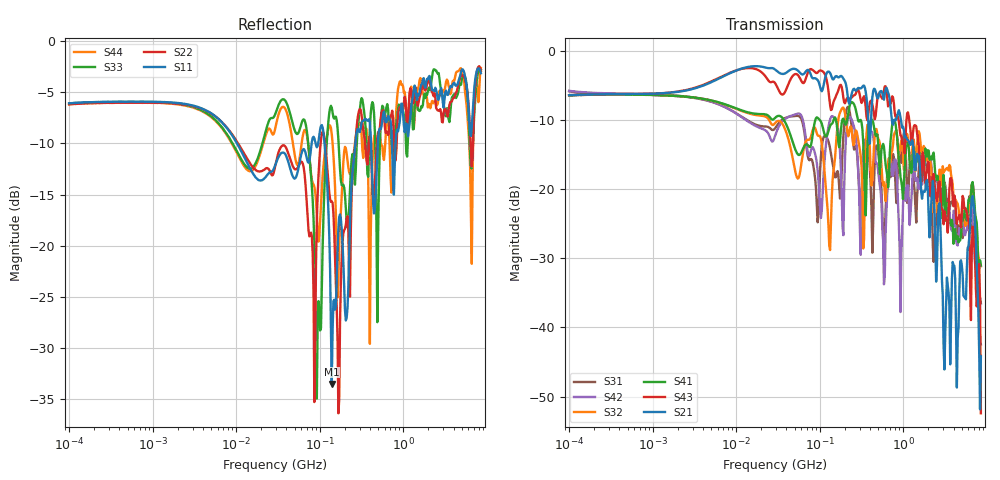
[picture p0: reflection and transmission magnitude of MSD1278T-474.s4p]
# MHz S MA R 50
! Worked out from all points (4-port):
!   498 points, 100 kHz to 8.5 GHz, reference 50 ohm
!   strongest paths, dB at 100 kHz, 1.698 MHz, 29.49 MHz, 500.7 MHz, 8.5 GHz:
!     S21: -6.3, -6.0, -2.7, -6.8, -44.2
!     S43: -6.3, -5.9, -4.7, -6.2, -52.4
!     S41: -6.4, -6.4, -9.6, -13.2, -31.0
!     S32: -6.4, -6.4, -10.3, -12.6, -31.1
!     S42: -5.7, -6.4, -12.1, -17.4, -42.4
!     S31: -5.8, -6.4, -11.1, -14.3, -36.5
!   lowest |S11| = -33.5 dB at 139.4 MHz (marker M1), VSWR 1.04, Z = 49.2 - j1.95 ohm
!   |S11| at or under -10 dB: 10.23 MHz to 80.11 MHz (69.88 MHz wide, 155 % of centre); 114.2 MHz to 267.3 MHz (153.1 MHz wide, 80.3 % of centre); 411.1 MHz to 496.6 MHz (85.5 MHz wide, 18.8 % of centre)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
0.1  0.4965 9.5  0.4816 10.7  0.5139 -10.4  0.4796 -170.7
     0.4816 10.7  0.491 9.5  0.4794 -170.6  0.5185 -10.4
     0.5139 -10.4  0.4794 -170.6  0.4954 9.6  0.4817 10.6
     0.4796 -170.7  0.5185 -10.4  0.4817 10.6  0.4895 9.7
37.91146  0.2831 -18.0  0.6897 -8.1  0.328 143.2  0.3131 -14.9
          0.6897 -8.1  0.3081 -21.9  0.2793 -13.7  0.3218 140.6
          0.328 143.2  0.2793 -13.7  0.516 -21.2  0.5011 -2.1
          0.3131 -14.9  0.3218 140.6  0.5011 -2.1  0.4724 -22.7
94.51579  0.307 -42.1  0.6194 -27.6  0.05783 27.1  0.3304 61.7
          0.6194 -27.6  0.1778 51.5  0.2463 17.5  0.1368 -51.7
          0.05783 27.1  0.2463 17.5  0.04302 2.5  0.7036 -23.4
          0.3304 61.7  0.1368 -51.7  0.7036 -23.4  0.1177 -47.5
139.353  0.02113 -110.7  0.6498 -33.4  0.1669 -10.5  0.2983 27.8
         0.6498 -33.4  0.1651 -55.2  0.0868 77.1  0.3393 27.6
         0.1669 -10.5  0.0868 77.1  0.4728 -13.7  0.3785 -34.4
         0.2983 27.8  0.3393 27.6  0.3785 -34.4  0.3516 -78.4
2365.873  0.57 169.9  0.06787 39.1  0.04002 134.4  0.1553 85.9
          0.06787 39.1  0.5554 160.1  0.095 120.1  0.1206 112.8
          0.04002 134.4  0.095 120.1  0.727 171.6  0.1128 82.0
          0.1553 85.9  0.1206 112.8  0.1128 82.0  0.4959 173.8
6764.496  0.4391 48.9  0.08958 5.4  0.04947 25.2  0.1131 59.7
          0.08958 5.4  0.281 84.7  0.1122 50.7  0.05657 30.6
          0.04947 25.2  0.1122 50.7  0.2842 48.7  0.05377 -10.1
          0.1131 59.7  0.05657 30.6  0.05377 -10.1  0.209 53.4
8500  0.6964 -59.3  0.006163 -8.6  0.01495 -103.0  0.02811 -120.9
      0.006163 -8.6  0.7146 -57.4  0.02778 -121.8  0.007543 -110.1
      0.01495 -103.0  0.02778 -121.8  0.7232 -53.8  0.002389 86.9
      0.02811 -120.9  0.007543 -110.1  0.002389 86.9  0.7382 -44.4
